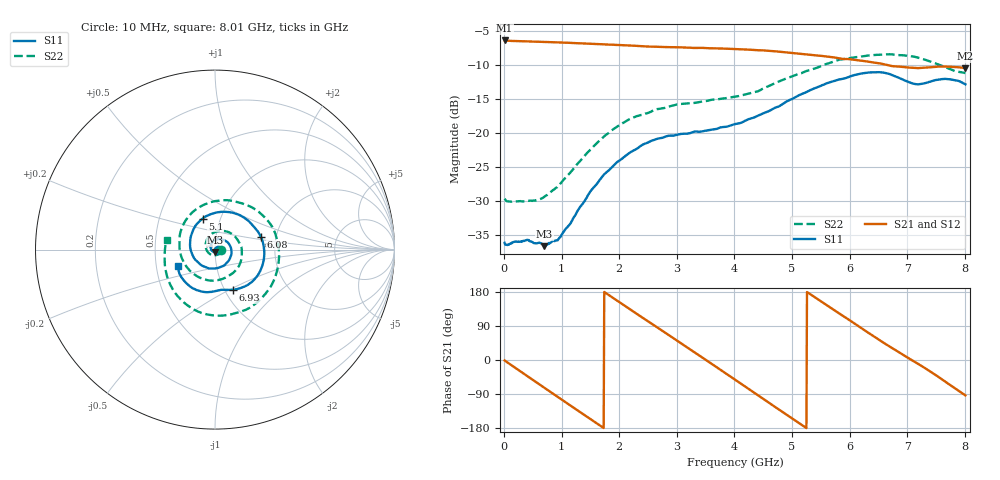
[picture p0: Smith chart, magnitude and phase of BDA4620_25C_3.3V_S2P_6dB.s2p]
!Agilent Technologies,E5071B,MY42404982,A.09.10
!Date: Wed May 06 08:49:35 2026
!Data & Calibration Information:
!Freq	S11:SOLT2(ON)	S21:SOLT2(ON)	S12:SOLT2(ON)	S22:SOLT2(ON)
# Hz S RI R 50
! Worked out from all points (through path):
!   801 points, 10 MHz to 8.01 GHz, reference 50 ohm
!   highest |S21| = -6.44 dB at 10 MHz (marker M1); lowest = -10.5 dB at 8.01 GHz (marker M2)
!   group delay of S21, straight-line fit = 282 ps
!   lowest |S11| = -36.7 dB at 700 MHz (marker M3), VSWR 1.03, Z = 50.1 - j1.46 ohm
!   |S11| at or under -10 dB: start of sweep to end of sweep
!   |S22| runs from -30.2 to -8.5 dB; largest |S21 - S12| = 0.0019
!   S11 on the Smith chart (normalised r, x): 10 MHz: 1.03, -0.00; 5.1 GHz: 0.82, +0.29; 6.08 GHz: 1.66, +0.26; 6.93 GHz: 1.09, -0.52; 8.01 GHz: 0.65, -0.12
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1e7  0.0154 -0.000917  0.4764 -0.0101  0.4768 -0.0101  0.0326 -0.00248
3.3e8  0.0136 -0.00828  0.386 -0.2682  0.3866 -0.2687  0.0208 -0.0233
7e8  0.00144 -0.0145  0.1339 -0.4452  0.1338 -0.4459  -0.012 -0.0315
1.01e9  -0.016 -0.00811  -0.1218 -0.4433  -0.1221 -0.4438  -0.0426 -0.0103
1.35e9  -0.0248 0.016  -0.35 -0.2887  -0.3502 -0.289  -0.051 0.0385
1.64e9  -0.0139 0.0414  -0.4414 -0.0761  -0.4418 -0.0761  -0.0252 0.0821
1.93e9  0.0138 0.0573  -0.4157 0.1505  -0.4162 0.151  0.0286 0.1045
2.32e9  0.061 0.0468  -0.2184 0.3755  -0.219 0.3757  0.1101 0.0743
2.68e9  0.0905 0.00412  0.045 0.4255  0.0456 0.4258  0.1493 -0.00232
3e9  0.084 -0.0468  0.2644 0.3324  0.2646 0.3325  0.136 -0.0863
3.39e9  0.0394 -0.0936  0.411 0.0864  0.4114 0.086  0.0487 -0.1605
3.69e9  -0.0141 -0.1057  0.3943 -0.1345  0.3939 -0.1353  -0.0509 -0.168
4.01e9  -0.0763 -0.0866  0.2547 -0.3242  0.2546 -0.3248  -0.1497 -0.107
4.52e9  -0.1387 0.017  -0.1011 -0.3892  -0.1017 -0.3895  -0.195 0.0862
5.1e9  -0.0691 0.1729  -0.3675 -0.1031  -0.3683 -0.102  -0.00472 0.2693
5.35e9  0.0134 0.208  -0.3669 0.0629  -0.3669 0.0634  0.12 0.266
5.73e9  0.1579 0.1807  -0.2369 0.2678  -0.2366 0.2684  0.2898 0.1655
6.08e9  0.2548 0.0726  -0.0396 0.3414  -0.0387 0.3418  0.357 -0.0223
6.68e9  0.194 -0.1893  0.2503 0.1869  0.2513 0.1869  0.1987 -0.3205
6.93e9  0.1001 -0.2239  0.2956 0.0713  0.2965 0.0705  0.056 -0.3664
7.48e9  -0.0542 -0.2368  0.2388 -0.1886  0.239 -0.1897  -0.2316 -0.2276
8.01e9  -0.2081 -0.09  -0.018 -0.2974  -0.0187 -0.2984  -0.2689 0.0537
